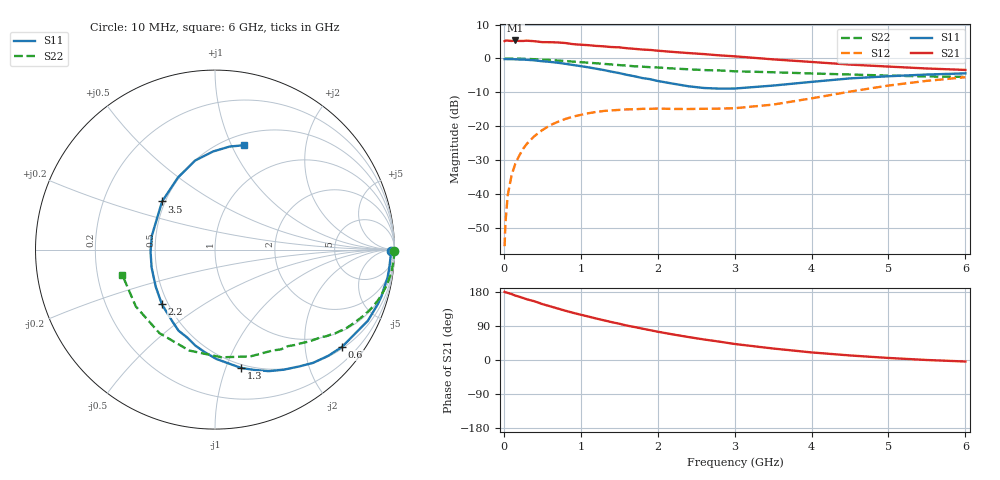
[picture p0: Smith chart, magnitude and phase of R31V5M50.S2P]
! SIEMENS Small Signal Semiconductors
! BFR181
! Si NPN RF Bipolar Junction Transistor in SOT23
! VCE = 1.5 V  IC = 0.5 mA
! Common Emitter S-Parameters:  May  1996
# GHz  S  MA  R  50
!  f  S11  S21  S12  S22
! GHz  MAG  ANG  MAG  ANG  MAG  ANG  MAG  ANG
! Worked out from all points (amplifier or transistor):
!   36 points, 10 MHz to 6 GHz, reference 50 ohm
!   highest |S21| = 5.3 dB at 150 MHz (marker M1)
!   |S21| within 3 dB of that: start of sweep to 1.991 GHz
!   unconditionally stable (mu >= 1): 2.324 GHz to 4.044 GHz
!   at 250 MHz: K = 0.13, MSG = 15.9 dB, |S12| = -26.7 dB
!   at 1.4 GHz: K = 0.62, MSG = 9.3 dB, |S12| = -15.3 dB
!   at 6 GHz: K = 0.94, MSG = 1.1 dB, |S12| = -5.5 dB
!   S11 on the Smith chart (normalised r, x): 10 MHz: 74, -35; 600 MHz: 0.54, -2.86; 1.3 GHz: 0.47, -1.13; 2.2 GHz: 0.46, -0.34; 3.5 GHz: 0.48, +0.31; 6 GHz: 0.61, +1.12
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0.01  0.9783 -0.6  1.808 179.8  0.0017 90.0  0.9999 -0.3
0.02  0.9803 -1.1  1.839 178.7  0.0036 91.9  0.9943 -0.6
0.05  0.9783 -3.1  1.835 177.1  0.0095 87.9  0.9984 -1.5
0.1  0.9765 -6.1  1.814 174.1  0.0188 85.7  0.9975 -2.9
0.15  0.974 -9.3  1.846 169.9  0.0282 83.0  0.9943 -4.5
0.3  0.9566 -18.6  1.833 160.2  0.0553 77.0  0.9857 -9.0
0.6  0.8914 -37.4  1.74 141.8  0.1034 64.8  0.9509 -17.3
0.8  0.8348 -49.1  1.691 130.0  0.1282 57.1  0.9175 -22.3
1.1  0.7407 -66.1  1.572 114.6  0.1557 48.0  0.8665 -29.0
1.3  0.6748 -77.6  1.51 104.8  0.1682 42.7  0.833 -32.9
1.5  0.609 -89.4  1.462 95.7  0.1742 38.8  0.7991 -36.4
1.6  0.5737 -95.8  1.417 90.8  0.1775 36.8  0.7855 -37.9
2  0.4661 -120.5  1.304 74.7  0.1826 32.6  0.7367 -43.8
2.2  0.425 -134.1  1.25 67.4  0.1801 32.1  0.7118 -47.0
2.6  0.3671 -164.2  1.162 54.2  0.1811 34.0  0.6745 -52.9
3  0.3603 167.8  1.077 42.3  0.1846 38.2  0.6475 -60.2
3.5  0.3985 137.7  0.971 30.3  0.2088 44.7  0.6269 -71.7
4  0.4519 117.1  0.889 20.0  0.2581 48.9  0.6011 -86.6
4.5  0.5087 102.5  0.813 12.0  0.3246 47.7  0.5804 -104.3
5  0.5469 91.1  0.76 5.4  0.399 42.6  0.559 -123.6
5.5  0.5799 81.9  0.712 0.0  0.4683 35.2  0.5431 -144.3
6  0.6036 74.4  0.678 -4.0  0.529 26.6  0.5355 -164.9
